(* Logix 5000 DataType export AMCI_5034_PTO_AM_Input_Data; software revision 37.00 *)

TYPE AMCI_5034_PTO_AM_Input_Data :
STRUCT
   ConnectionFaulted : DINT;
   MovingCW : BOOL;
   MovingCCW : BOOL;
   InHoldState : BOOL;
   Stopped : BOOL;
   AtHome : BOOL;
   Accelerating : BOOL;
   Decelerating : BOOL;
   MoveComplete : BOOL;
   HomeInvalid : BOOL;
   InvalidProfile : BOOL;
   PositionInvalid : BOOL;
   InputError : BOOL;
   CommandError : BOOL;
   ConfigurationError : BOOL;
   ModuleOK : BOOL;
   GeneralPurposeOutputStatus : BOOL;
   Input1Active : BOOL;
   Input2Active : BOOL;
   Input3Active : BOOL;
   Input4Active : BOOL;
   bit_20_reserved : BOOL;
   bit_21_reserved : BOOL;
   bit_22_reserved : BOOL;
   EncoderFollowerMode : BOOL;
   BlendMoveRunning : BOOL;
   BlendMoveAcknowledge : BOOL;
   MinimumRegistrationProgrammed : BOOL;
   EncoderMotionDirection : BOOL;
   MultipleInputsWithSameFunction : BOOL;
   FSCExceedsNumberOfDataBits : BOOL;
   AbsoluteEncoderSetupError : BOOL;
   bit_31_reserved : BOOL;
   CurrentPosition : DINT;
   EncoderPosition : DINT;
   CapturedPosition : DINT;
END_STRUCT
END_TYPE
